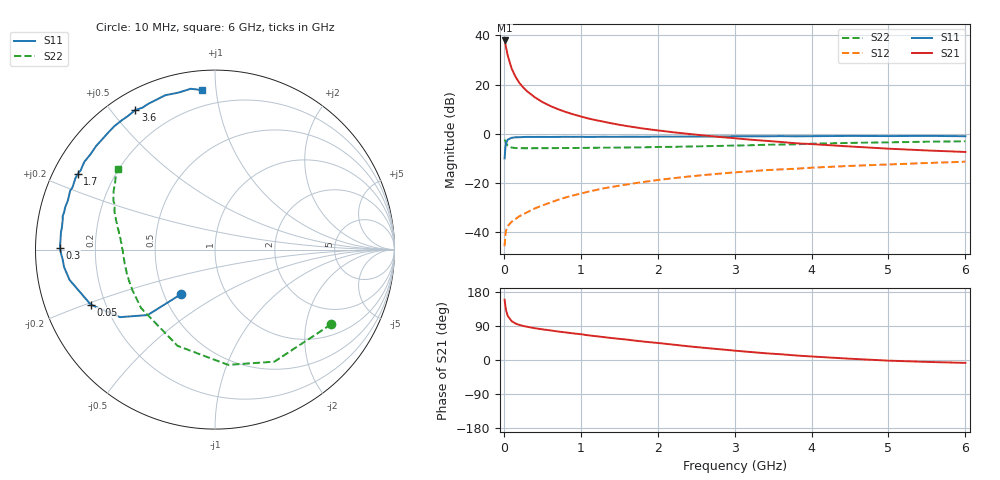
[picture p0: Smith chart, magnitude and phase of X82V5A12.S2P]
! SIEMENS Small Signal Semiconductors
! BFP136W
! Si NPN RF Bipolar Junction Transistor in SOT343
! VCE = 2.5 V  IC = 120 mA
! Common Emitter S-Parameters:  September  1994
# GHz  S  MA  R  50
!  f  S11  S21  S12  S22
! GHz  MAG  ANG  MAG  ANG  MAG  ANG  MAG  ANG
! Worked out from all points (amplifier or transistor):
!   40 points, 10 MHz to 6 GHz, reference 50 ohm
!   highest |S21| = 37.9 dB at 10 MHz (marker M1)
!   |S21| within 3 dB of that: start of sweep to 29.85 MHz
!   unconditionally stable (mu >= 1): 475.8 MHz to 2.937 GHz
!   at 200 MHz: K = 0.73, MSG = 27.2 dB, |S12| = -33.6 dB
!   at 1.5 GHz: K = 1.11, MAG = 10.4 dB, |S12| = -21.1 dB
!   at 6 GHz: K = 0.98, MSG = 2.0 dB, |S12| = -11.3 dB
!   S11 on the Smith chart (normalised r, x): 10 MHz: 0.61, -0.34; 50 MHz: 0.14, -0.21; 300 MHz: 0.07, +0.01; 1.7 GHz: 0.07, +0.26; 3.6 GHz: 0.07, +0.58; 6 GHz: 0.11, +0.92
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0.01  0.3153 -127.5  78.75 159.3  0.0052 68.5  0.7698 -32.7
0.02  0.5231 -135.8  66.83 142.2  0.0089 55.9  0.7066 -62.1
0.03  0.6497 -144.6  55.59 130.4  0.0111 48.8  0.6464 -83.5
0.05  0.757 -156.1  39.17 116.6  0.0133 39.3  0.5755 -111.2
0.1  0.8275 -168.2  21.45 102.7  0.0162 39.2  0.5252 -141.6
0.15  0.8465 -173.4  14.56 96.5  0.0185 41.7  0.5127 -153.9
0.2  0.8504 -176.2  10.93 92.7  0.021 43.9  0.5093 -160.4
0.25  0.8588 -178.8  8.811 89.9  0.0231 47.3  0.5091 -164.6
0.3  0.8641 179.4  7.367 87.8  0.0252 50.4  0.5079 -167.4
0.4  0.8624 176.2  5.551 84.0  0.0303 53.9  0.509 -171.2
0.5  0.8636 173.6  4.422 80.9  0.0349 57.2  0.5099 -173.9
0.6  0.862 171.8  3.691 78.3  0.0398 58.8  0.5106 -175.6
0.8  0.8687 167.6  2.787 72.9  0.0506 61.3  0.5132 -178.2
1.1  0.8642 161.6  2.041 65.0  0.0665 62.0  0.5178 178.9
1.4  0.8664 156.6  1.63 58.0  0.083 61.5  0.5217 176.5
1.7  0.8732 151.1  1.359 51.2  0.0988 59.7  0.5287 174.0
2.2  0.8738 142.7  1.074 40.6  0.1249 55.6  0.5423 170.2
3.2  0.888 125.8  0.76 21.2  0.1727 45.9  0.5842 161.4
3.6  0.8959 119.7  0.682 15.2  0.1889 42.0  0.6041 157.9
4.5  0.9036 107.8  0.552 3.4  0.2222 33.3  0.6523 150.0
5.5  0.9063 98.6  0.458 -5.0  0.2545 25.5  0.6897 143.3
6  0.8911 94.5  0.427 -7.6  0.2709 21.1  0.7039 140.4
